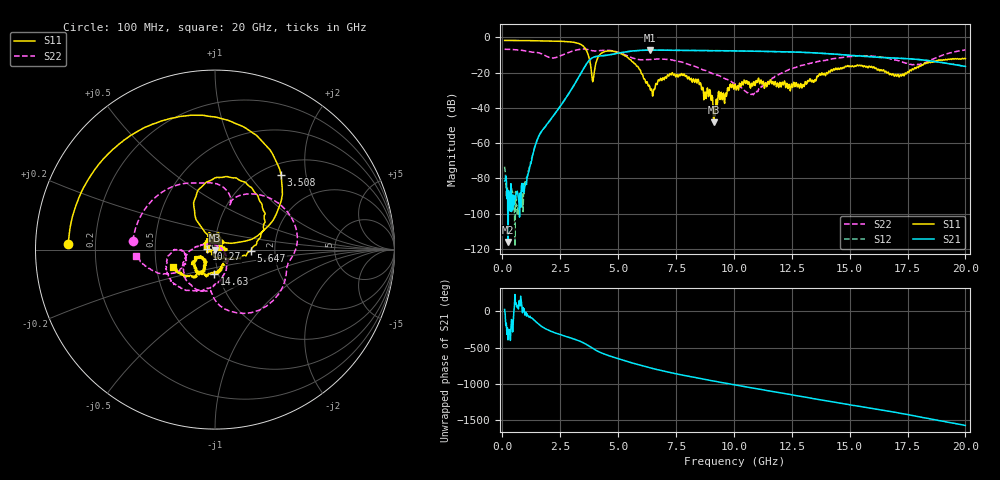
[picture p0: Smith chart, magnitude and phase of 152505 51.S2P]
!  2-Port S-parameters saved by WinCal
! VAR MeasName=S-Parameters (CALIBRATED_DATA) read from VNA (N5230C)
! VAR MeasDate=4/10/2015 9:33:42 AM
! VAR NAME=152505 51
! VAR FILENAME=152505 51.S2P
! VAR DATE=4/10/2015 9:33:42 AM
! VAR PHYS_PORTS=1,2
# Hz S DB R 50
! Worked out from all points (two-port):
!   801 points, 100 MHz to 20 GHz, reference 50 ohm
!   highest |S21| = -7.20 dB at 6.393 GHz (marker M1); lowest = -116.1 dB at 249.2 MHz (marker M2)
!   |S21| within 3 dB of the highest: 4.468 GHz to 15.02 GHz (10.55 GHz wide, 108 % of centre); 15.04514 GHz to 15.0544 GHz (9.257 MHz wide, 0.0615 % of centre)
!   lowest |S11| = -48.1 dB at 9.13 GHz (marker M3), VSWR 1.01, Z = 49.9 - j0.366 ohm
!   |S11| at or under -10 dB: 3.714 GHz to 4.204 GHz (490.9 MHz wide, 12.4 % of centre); 5.252 GHz to end of sweep
!   |S22| runs from -32.5 to -6.6 dB; largest |S21 - S12| = 0.0054
!   S11 on the Smith chart (normalised r, x): 100 MHz: 0.10, +0.02; 3.508 GHz: 1.21, +1.46; 5.647 GHz: 1.50, -0.03; 10.27 GHz: 0.91, +0.01; 14.63 GHz: 0.95, -0.27; 20 GHz: 0.61, -0.12
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1e8  -1.75 177.6  -81.44 25.9  -73.33 96.6  -6.75 173.9
2.4925e8  -1.75 174.1  -116.09 -33.4  -90.27 39.8  -6.78 164.6
1.04525e9  -1.83 154.9  -83.45 -65.3  -79.41 -26.6  -7.78 116.0
1.5925e9  -1.92 140.9  -55.68 178.3  -55.55 178.1  -8.82 86.6
3.43325e9  -4.33 56.8  -19.48 -64.1  -19.53 -64.1  -6.67 20.0
3.507875e9  -5.10 48.5  -17.81 -75.7  -17.83 -75.8  -6.62 14.3
3.905875e9  -25.13 63.4  -11.46 -153.0  -11.48 -153.0  -7.60 -9.5
4.453125e9  -7.91 88.8  -10.24 123.9  -10.32 123.5  -7.28 -35.3
5.647125e9  -13.97 -2.4  -7.66 2.6  -7.69 2.6  -11.75 -92.5
6.393375e9  -29.88 -105.1  -7.20 -62.5  -7.23 -62.5  -12.55 -102.5
6.741625e9  -24.07 155.7  -7.24 -89.4  -7.23 -89.7  -12.22 -113.9
7.861e9  -20.79 79.3  -7.43 -166.5  -7.40 -166.3  -14.44 -158.4
8.9555e9  -29.59 -6.5  -7.55 125.9  -7.55 126.1  -19.82 169.5
9.129625e9  -48.11 -110.8  -7.56 115.7  -7.53 115.7  -20.87 169.1
1.005e10  -26.55 -170.3  -7.67 62.1  -7.68 62.1  -26.42 137.7
1.027388e10  -26.68 175.3  -7.73 49.7  -7.74 49.7  -28.23 128.3
1.0846e10  -25.40 143.5  -7.85 17.4  -7.82 17.6  -32.49 57.5
1.338325e10  -24.33 -9.4  -8.75 -123.6  -8.74 -123.4  -14.40 -87.9
1.4627e10  -17.28 -92.1  -9.80 167.8  -9.81 167.5  -11.52 -121.1
1.669162e10  -20.28 -150.2  -11.57 57.9  -11.56 57.4  -11.95 -173.9
1.79105e10  -16.72 -119.1  -12.44 -12.5  -12.51 -12.9  -15.58 -164.2
2e10  -11.99 -157.8  -16.51 -138.5  -16.49 -138.1  -7.10 -175.6
